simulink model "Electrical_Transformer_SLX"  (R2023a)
settings: Solver=ode23s  StartTime=0.0  StopTime=10.0  MaxStep=0.001  RelTol=1e-3
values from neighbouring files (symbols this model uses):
  C_3 = 0.001*F    (= 0.001)    [Electrical_Transformer_EQN.m]    (also in Electrical_Transformer_SLX_m.m; BIG_EC_Simscape_EQN.m; BIG_EC_Simscape_SLX_m.m; Electric_Circuit_03_EQN.m)
  C_7 = 0.001*F    (= 0.001)    [Electrical_Transformer_EQN.m]    (also in Electrical_Transformer_SLX_m.m; Electric_Circuit_02_EQN.m; Electric_Circuit_02_SLX_m.m; Electric_Circuit_04_EQN.m)
  I_2_0 = 0*A    (= 0)    [Electrical_Transformer_SLX_m.m]    (also in Electric_Circuit_02_SLX_m.m; Electric_Circuit_03_SLX_m.m; Electric_Circuit_06_SLX_m.m; Electric_Circuit_08_SLX_m.m)
  I_8_0 = 0*A    (= 0)    [Electrical_Transformer_SLX_m.m]    (also in Electric_Circuit_02_SLX_m.m; Electric_Circuit_05_SLX_m.m; Electric_Circuit_06_SLX_m.m; Electric_Circuit_07_SLX_m.m)
  L_2 = 0.002*H    (= 0.002)    [Electrical_Transformer_EQN.m]    (also in Electrical_Transformer_SLX_m.m; Electric_Circuit_02_EQN.m; Electric_Circuit_02_SLX_m.m; Electric_Circuit_03_EQN.m)
  L_8 = 0.002*H    (= 0.002)    [Electrical_Transformer_EQN.m]    (also in Electrical_Transformer_SLX_m.m)
  R = 1    [Electrical_Transformer_EQN.m]    (also in Electrical_Transformer_SLX_m.m; Mechanical_Transmission_EQN.m; Mechanical_Transmission_SLX_m.m; Mechanical_system_EQN.m)
  R_4 = 100*Ohm    (= 100)    [Electrical_Transformer_EQN.m]    (also in Electrical_Transformer_SLX_m.m; BIG_EC_Simscape_EQN.m; BIG_EC_Simscape_SLX_m.m; Electric_Circuit_08_EQN.m)
  Ts = Tfin/Nr_Ts_Points    (= 0.0005999)    [Electrical_Transformer_SLX_m.m]    (also in BIG_EC_Simscape_SLX_m.m = 0.0003; Car_Dumper_SLX_m.m = 0.0022779; Electric_Circuit_01_SLX_m.m = 0.005; Electric_Circuit_02_SLX_m.m = 0.000480145)
  V_1_0 = 10*V    (= 10)    [Electrical_Transformer_SLX_m.m]    (also in BIG_EC_Simscape_SLX_m.m; Electric_Circuit_02_SLX_m.m; Electric_Circuit_03_SLX_m.m; Electric_Circuit_04_SLX_m.m)
  V_3_0 = 0*V    (= 0)    [Electrical_Transformer_SLX_m.m]    (also in BIG_EC_Simscape_SLX_m.m; Electric_Circuit_03_SLX_m.m; Electric_Circuit_07_SLX_m.m; Electric_Circuit_11_SLX_m.m)
  V_7_0 = 0*V    (= 0)    [Electrical_Transformer_SLX_m.m]    (also in Electric_Circuit_02_SLX_m.m; Electric_Circuit_04_SLX_m.m; Electric_Circuit_05_SLX_m.m; Electric_Circuit_07_SLX_m.m)
  V_9_0 = 0*V    (= 0)    [Electrical_Transformer_SLX_m.m]

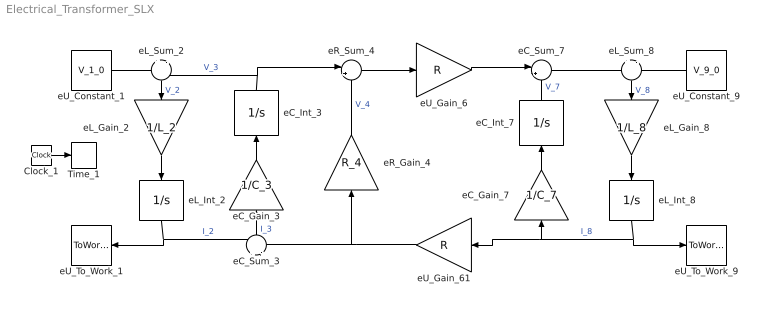
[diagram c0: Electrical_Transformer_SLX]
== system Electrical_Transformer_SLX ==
  Clock_1 : Clock
  Time_1 : ToWorkspace  VariableName=t  SaveFormat=Timeseries  SampleTime=Ts
  eC_Gain_3 : Gain  Gain=1/C_3  Multiplication=Matrix(K*u)
  eC_Gain_7 : Gain  Gain=1/C_7  Multiplication=Matrix(K*u)
  eC_Int_3 : Integrator  InitialCondition=V_3_0
  eC_Int_7 : Integrator  InitialCondition=V_7_0
  eC_Sum_3 : Sum  Inputs=+|-
  eC_Sum_7 : Sum  Inputs=|+-
  eL_Gain_2 : Gain  Gain=1/L_2  Multiplication=Matrix(K*u)
  eL_Gain_8 : Gain  Gain=1/L_8  Multiplication=Matrix(K*u)
  eL_Int_2 : Integrator  InitialCondition=I_2_0
  eL_Int_8 : Integrator  InitialCondition=I_8_0
  eL_Sum_2 : Sum  Inputs=+|-
  eL_Sum_8 : Sum  Inputs=+|-
  eR_Gain_4 : Gain  Gain=R_4  Multiplication=Matrix(K*u)
  eR_Sum_4 : Sum  Inputs=|+-
  eU_Constant_1 : Constant  Value=V_1_0
  eU_Constant_9 : Constant  Value=V_9_0
  eU_Gain_6 : Gain  Gain=R  Multiplication=Matrix(K*u)
  eU_Gain_61 : Gain  Gain=R  Multiplication=Matrix(K*u)
  eU_To_Work_1 : ToWorkspace  VariableName=I_1_0  SaveFormat=Timeseries  SampleTime=Ts
  eU_To_Work_9 : ToWorkspace  VariableName=I_9_0  SaveFormat=Timeseries  SampleTime=Ts
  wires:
  eU_Constant_1/1 -> eL_Sum_2/1
  eC_Int_3/1 -> eL_Sum_2/2, eR_Sum_4/1  "V_3"
  eL_Int_2/1 -> eU_To_Work_1/1, eC_Sum_3/1  "I_2"
  eL_Sum_2/1 -> eL_Gain_2/1  "V_2"
  eL_Gain_2/1 -> eL_Int_2/1
  eU_Gain_61/1 -> eC_Sum_3/2, eR_Gain_4/1
  eC_Sum_3/1 -> eC_Gain_3/1  "I_3"
  eC_Gain_3/1 -> eC_Int_3/1
  eR_Sum_4/1 -> eU_Gain_6/1
  eR_Gain_4/1 -> eR_Sum_4/2  "V_4"
  eU_Gain_6/1 -> eC_Sum_7/1
  eL_Int_8/1 -> eU_Gain_61/1, eC_Gain_7/1, eU_To_Work_9/1  "I_8"
  eC_Sum_7/1 -> eL_Sum_8/1
  eC_Gain_7/1 -> eC_Int_7/1
  eC_Int_7/1 -> eC_Sum_7/2  "V_7"
  eU_Constant_9/1 -> eL_Sum_8/2
  eL_Sum_8/1 -> eL_Gain_8/1  "V_8"
  eL_Gain_8/1 -> eL_Int_8/1
  Clock_1/1 -> Time_1/1
